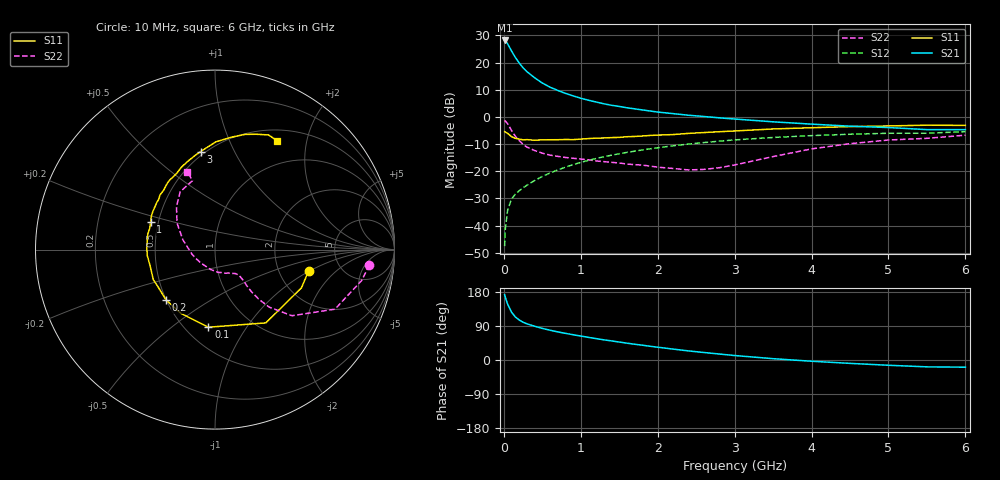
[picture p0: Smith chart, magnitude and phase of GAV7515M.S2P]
! Infineon Technologies  Discrete & RF Semiconductors
! BF775
! Si NPN RF Bipolar Junction Transistor in SOT23
! VCE = 0.75 V  IC = 15 mA
! Common Emitter S-Parameters:  May  1996
# GHz  S  MA  R  50
!  f  S11  S21  S12  S22
! GHz  MAG  ANG  MAG  ANG  MAG  ANG  MAG  ANG
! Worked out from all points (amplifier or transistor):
!   36 points, 10 MHz to 6 GHz, reference 50 ohm
!   highest |S21| = 28.1 dB at 10 MHz (marker M1)
!   |S21| within 3 dB of that: start of sweep to 83.38 MHz
!   unconditionally stable (mu >= 1): 228 MHz to end of sweep
!   at 250 MHz: K = 1.05, MAG = 20.7 dB, |S12| = -26.1 dB
!   at 1.4 GHz: K = 1.36, MAG = 5.6 dB, |S12| = -14.1 dB
!   at 6 GHz: K = 1.11, MAG = -1.7 dB, |S12| = -5.4 dB
!   S11 on the Smith chart (normalised r, x): 10 MHz: 2.95, -0.97; 100 MHz: 0.64, -0.69; 200 MHz: 0.50, -0.33; 1 GHz: 0.45, +0.17; 3 GHz: 0.47, +0.74; 6 GHz: 0.64, +1.53
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0.01  0.5351 -12.7  25.48 172.5  0.0042 81.7  0.864 -5.7
0.02  0.5266 -23.9  24.94 165.3  0.0089 77.8  0.8359 -11.8
0.05  0.4967 -55.3  22.02 147.1  0.0196 68.3  0.7464 -26.4
0.1  0.4339 -94.8  16.33 126.1  0.0309 58.0  0.565 -40.7
0.15  0.4028 -118.3  12.41 113.5  0.038 55.9  0.4404 -46.7
0.2  0.3911 -134.4  9.82 105.6  0.0439 56.3  0.3667 -48.6
0.25  0.3792 -146.3  8.002 99.7  0.0496 56.9  0.3128 -49.1
0.3  0.3824 -154.0  6.803 95.5  0.0555 59.2  0.2791 -48.9
0.4  0.3726 -166.1  5.248 89.1  0.0677 61.1  0.241 -47.7
0.5  0.379 -175.1  4.203 83.4  0.0803 62.6  0.2156 -47.1
0.6  0.3803 177.9  3.527 78.6  0.093 63.4  0.1985 -47.0
0.7  0.3808 171.6  3.075 74.2  0.1058 63.3  0.1882 -47.9
0.8  0.3844 167.0  2.715 70.4  0.1191 62.9  0.1797 -48.9
1  0.3907 156.6  2.209 63.2  0.1456 61.9  0.1684 -51.9
1.1  0.4001 152.5  2.028 59.7  0.1588 61.0  0.1627 -54.9
1.6  0.4322 135.2  1.473 44.4  0.2227 55.2  0.1361 -71.4
2.2  0.4737 117.2  1.15 28.8  0.2943 46.8  0.1129 -103.9
3  0.5518 98.4  0.915 11.8  0.3779 34.6  0.1307 -168.5
3.5  0.6007 89.5  0.813 3.5  0.4189 26.9  0.1865 163.3
4.5  0.6634 75.4  0.676 -8.9  0.4806 12.7  0.3225 131.7
5.5  0.7049 65.0  0.584 -18.1  0.5017 -0.7  0.404 108.1
6  0.6989 60.2  0.584 -19.0  0.5353 -4.6  0.4614 109.5
